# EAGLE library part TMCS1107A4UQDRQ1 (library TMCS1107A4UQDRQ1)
TMCS1107A4UQDRQ1 Source: Datasheet
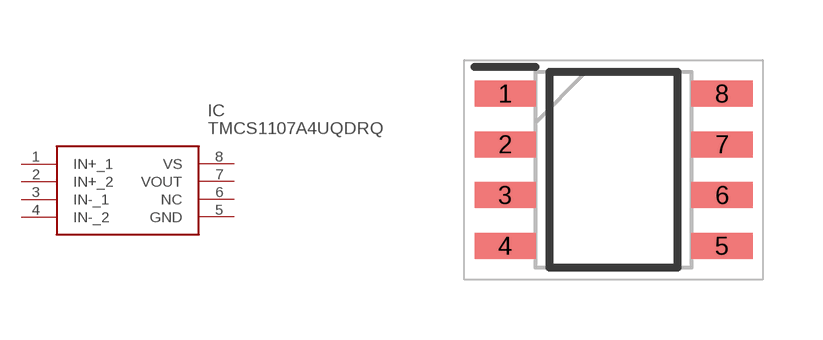
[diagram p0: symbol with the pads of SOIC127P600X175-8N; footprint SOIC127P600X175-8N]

Designator prefix IC

## TMCS1107A4UQDRQ1 (Description: TMCS1107A4UQDRQ1; Height: 1.75mm; Manufacturer_Name: Texas Instruments; Manufacturer_Part_Number: TMCS1107A4UQDRQ1; Mouser_Part_Number: 595-TMCS1107A4UQDRQ1; Mouser_Price-Stock: https://www.mouser.co.uk/ProductDetail/Texas-Instruments/TMCS1107A4UQDRQ1?qs=A6eO%252BMLsxmQ8Ln0%2FPMa5pg%3D%3D)  [SOIC127P600X175-8N]
1  IN+_1
2  IN+_2
3  IN-_1
4  IN-_2
5  GND
6  NC  nc
7  VOUT
8  VS

## Footprint SOIC127P600X175-8N (pad centres in mm)
D
smd 1.528 x 0.65: 1 -2.711,1.905; 2 -2.711,0.635; 3 -2.711,-0.635; 4 -2.711,-1.905; 5 2.711,-1.905; 6 2.711,-0.635; 7 2.711,0.635; 8 2.711,1.905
